
FUNCTION_BLOCK FB4

TITLE =   <CALCULO DE DESVIACION DE TEMPERATURAS DEL MOTOR>
//

AUTHOR:   H3       //
FAMILY:   DESV     //
NAME:     FB_DESV  //
VERSION:  01.00    //
// KNOW_HOW_PROTECT


VAR_INPUT
  NUM_CILINDROS : INT;
  Promedio      : REAL; 	// PROMEDIO DE LA TEMPERATURA DE LOS CILINDROS
  Lim_desv_alto : REAL;     // LIMITE DE DESVIACION ALTO
  Lim_desv_bajo : REAL;	    // LIMITE DE DESVIACION BAJO

END_VAR



VAR

  	TEMP_CIL1	: REAL;
  	TEMP_CIL2	: REAL;
  	TEMP_CIL3	: REAL;
  	TEMP_CIL4	: REAL;
  	TEMP_CIL5	: REAL;
  	TEMP_CIL6	: REAL;
  	TEMP_CIL7	: REAL;
  	TEMP_CIL8	: REAL;
  	TEMP_CIL9	: REAL;
  	TEMP_CIL10	: REAL;
  	TEMP_CIL11	: REAL;
  	TEMP_CIL12	: REAL;
  	TEMP_CIL13	: REAL;
  	TEMP_CIL14	: REAL;
  	TEMP_CIL15	: REAL;
  	TEMP_CIL16	: REAL;
  	TEMP_CIL17	: REAL;
  	TEMP_CIL18	: REAL;
  	TEMP_CIL19	: REAL;
	TEMP_CIL20	: REAL;


  	DEV_CIL1	: REAL;
  	DEV_CIL2	: REAL;
  	DEV_CIL3	: REAL;
  	DEV_CIL4	: REAL;
  	DEV_CIL5	: REAL;
  	DEV_CIL6	: REAL;
  	DEV_CIL7	: REAL;
  	DEV_CIL8	: REAL;
  	DEV_CIL9	: REAL;
  	DEV_CIL10	: REAL;
  	DEV_CIL11	: REAL;
  	DEV_CIL12	: REAL;
  	DEV_CIL13	: REAL;
  	DEV_CIL14	: REAL;
  	DEV_CIL15	: REAL;
  	DEV_CIL16	: REAL;
  	DEV_CIL17	: REAL;
  	DEV_CIL18	: REAL;
  	DEV_CIL19	: REAL;
	DEV_CIL20	: REAL;


	DEV_CIL1_AL		: BOOL;
  	DEV_CIL2_AL		: BOOL;
  	DEV_CIL3_AL		: BOOL;
  	DEV_CIL4_AL		: BOOL;
  	DEV_CIL5_AL		: BOOL;
  	DEV_CIL6_AL		: BOOL;
  	DEV_CIL7_AL		: BOOL;
  	DEV_CIL8_AL		: BOOL;
  	DEV_CIL9_AL		: BOOL;
  	DEV_CIL10_AL	: BOOL;
  	DEV_CIL11_AL	: BOOL;
  	DEV_CIL12_AL	: BOOL;
  	DEV_CIL13_AL	: BOOL;
  	DEV_CIL14_AL	: BOOL;
  	DEV_CIL15_AL	: BOOL;
  	DEV_CIL16_AL	: BOOL;
  	DEV_CIL17_AL	: BOOL;
  	DEV_CIL18_AL	: BOOL;
  	DEV_CIL19_AL	: BOOL;
	DEV_CIL20_AL	: BOOL;


	FallSen_CIL1	: BOOL;
  	FallSen_CIL2	: BOOL;
  	FallSen_CIL3	: BOOL;
  	FallSen_CIL4	: BOOL;
  	FallSen_CIL5	: BOOL;
  	FallSen_CIL6	: BOOL;
  	FallSen_CIL7	: BOOL;
  	FallSen_CIL8	: BOOL;
  	FallSen_CIL9	: BOOL;
  	FallSen_CIL10	: BOOL;
  	FallSen_CIL11	: BOOL;
  	FallSen_CIL12	: BOOL;
  	FallSen_CIL13	: BOOL;
  	FallSen_CIL14	: BOOL;
  	FallSen_CIL15	: BOOL;
  	FallSen_CIL16	: BOOL;
  	FallSen_CIL17	: BOOL;
  	FallSen_CIL18	: BOOL;
  	FallSen_CIL19	: BOOL;
	FallSen_CIL20	: BOOL;

  	suma_temp : real;
  	num_cilindros_temp	: INT;


END_VAR


BEGIN
NETWORK
TITLE =   <VERIFICANDO FALLAD DE SENSOR>
// CALCULA EL PROMEDIO DE TEMPERATURA TOMANDO EN CUENTA
// LOS CILINDROS QUE PRESENTAN PROBLEMAS DE SENSOR Y LOS ELIMINA DEL
// CALCULO.
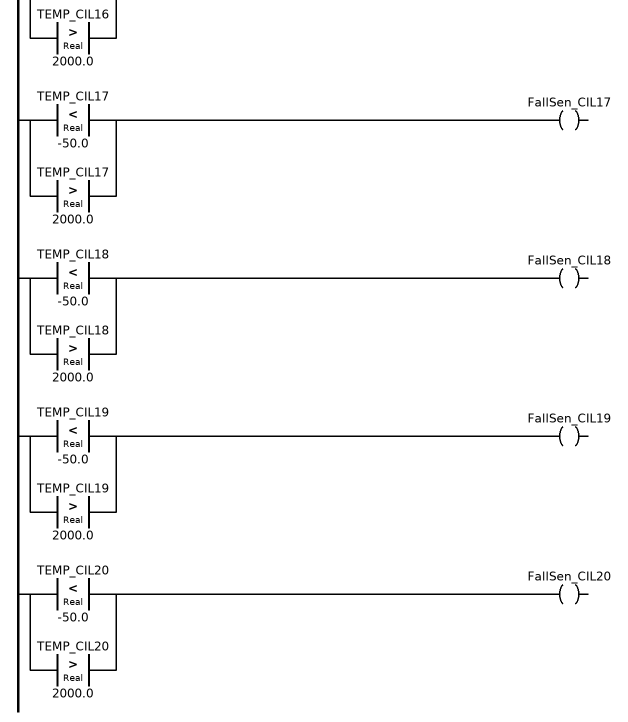
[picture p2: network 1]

	// Verificando falla de sensores
	O(;
	L TEMP_CIL1;
	L -50.0;
	<r;
	);
	o(;
	L TEMP_CIL1;
	L 2000.0;
	>r;
	);
	= FallSen_CIL1;

	O(;
	L TEMP_CIL2;
	L -50.0;
	<r;
	);
	o(;
	L TEMP_CIL2;
	L 2000.0;
	>r;
	);
	= FallSen_CIL2;

	O(;
	L TEMP_CIL3;
	L -50.0;
	<r;
	);
	o(;
	L TEMP_CIL3;
	L 2000.0;
	>r;
	);
	= FallSen_CIL3;


    O(;
	L TEMP_CIL4;
	L -50.0;
	<r;
	);
	o(;
	L TEMP_CIL4;
	L 2000.0;
	>r;
	);
	= FallSen_CIL4;

	O(;
	L TEMP_CIL4;
	L -50.0;
	<r;
	);
	o(;
	L TEMP_CIL4;
	L 2000.0;
	>r;
	);
	= FallSen_CIL4;


    O(;
	L TEMP_CIL5;
	L -50.0;
	<r;
	);
	o(;
	L TEMP_CIL5;
	L 2000.0;
	>r;
	);
	= FallSen_CIL5;


	O(;
	L TEMP_CIL6;
	L -50.0;
	<r;
	);
	o(;
	L TEMP_CIL6;
	L 2000.0;
	>r;
	);
	= FallSen_CIL6;


	O(;
	L TEMP_CIL7;
	L -50.0;
	<r;
	);
	o(;
	L TEMP_CIL7;
	L 2000.0;
	>r;
	);
	= FallSen_CIL7;


	O(;
	L TEMP_CIL8;
	L -50.0;
	<r;
	);
	o(;
	L TEMP_CIL8;
	L 2000.0;
	>r;
	);
	= FallSen_CIL8;

	O(;
	L TEMP_CIL9;
	L -50.0;
	<r;
	);
	o(;
	L TEMP_CIL9;
	L 2000.0;
	>r;
	);
	= FallSen_CIL9;


	O(;
	L TEMP_CIL10;
	L -50.0;
	<r;
	);
	o(;
	L TEMP_CIL10;
	L 2000.0;
	>r;
	);
	= FallSen_CIL10;


	O(;
	L TEMP_CIL11;
	L -50.0;
	<r;
	);
	o(;
	L TEMP_CIL11;
	L 2000.0;
	>r;
	);
	= FallSen_CIL11;

	O(;
	L TEMP_CIL12;
	L -50.0;
	<r;
	);
	o(;
	L TEMP_CIL12;
	L 2000.0;
	>r;
	);
	= FallSen_CIL12;


	O(;
	L TEMP_CIL13;
	L -50.0;
	<r;
	);
	o(;
	L TEMP_CIL13;
	L 2000.0;
	>r;
	);
	= FallSen_CIL13;


	O(;
	L TEMP_CIL14;
	L -50.0;
	<r;
	);
	o(;
	L TEMP_CIL14;
	L 2000.0;
	>r;
	);
	= FallSen_CIL14;


	O(;
	L TEMP_CIL15;
	L -50.0;
	<r;
	);
	o(;
	L TEMP_CIL15;
	L 2000.0;
	>r;
	);
	= FallSen_CIL15;


	O(;
	L TEMP_CIL16;
	L -50.0;
	<r;
	);
	o(;
	L TEMP_CIL16;
	L 2000.0;
	>r;
	);
	= FallSen_CIL16;


	O(;
	L TEMP_CIL17;
	L -50.0;
	<r;
	);
	o(;
	L TEMP_CIL17;
	L 2000.0;
	>r;
	);
	= FallSen_CIL17;


	O(;
	L TEMP_CIL18;
	L -50.0;
	<r;
	);
	o(;
	L TEMP_CIL18;
	L 2000.0;
	>r;
	);
	= FallSen_CIL18;


	O(;
	L TEMP_CIL19;
	L -50.0;
	<r;
	);
	o(;
	L TEMP_CIL19;
	L 2000.0;
	>r;
	);
	= FallSen_CIL19;

	O(;
	L TEMP_CIL20;
	L -50.0;
	<r;
	);
	o(;
	L TEMP_CIL20;
	L 2000.0;
	>r;
	);
	= FallSen_CIL20;

NETWORK
TITLE =   <CALCULA EL PROMEDIO DE LAS TEMPERATURAS>
// CALCULA EL PROMEDIO DE TEMPERATURA TOMANDO EN CUENTA

	L 0;
	T suma_temp;
  	L num_cilindros;
  	T num_cilindros_temp;


	L num_cilindros;
	L 1;
	<I;
	jc fin;

	AN FallSen_CIL1;
	jc cil1;

	L num_cilindros_temp;
	dec 1;
	T num_cilindros_temp;
	jc nxt2;

cil1:	L TEMP_CIL1;
	L suma_temp;
	+r;
	t suma_temp;


nxt2:	L num_cilindros;
	L 2;
	<I;
	jc fin;

	AN FallSen_CIL2;
	jc cil2;

	L num_cilindros_temp;
	dec 1;
	T num_cilindros_temp;
	jc nxt3;

cil2:	L TEMP_CIL2;
	L suma_temp;
	+r;
	t suma_temp;


nxt3:	L num_cilindros;
	L 3;
	<I;
	jc fin;

	AN FallSen_CIL3;
	jc cil3;

	L num_cilindros_temp;
	dec 1;
	T num_cilindros_temp;
	jc nxt4;

cil3:	L TEMP_CIL3;
	L suma_temp;
	+r;
	t suma_temp;


nxt4:	L num_cilindros;
	L 4;
	<I;
	jc fin;

	AN FallSen_CIL4;
	jc cil4;

	L num_cilindros_temp;
	dec 1;
	T num_cilindros_temp;
	jc nxt5;

cil4:	L TEMP_CIL4;
	L suma_temp;
	+r;
	t suma_temp;


nxt5:	L num_cilindros;
	L 5;
	<I;
	jc fin;

	AN FallSen_CIL5;
	jc cil5;

	L num_cilindros_temp;
	dec 1;
	T num_cilindros_temp;
	jc nxt6;

cil5:	L TEMP_CIL5;
	L suma_temp;
	+r;
	t suma_temp;


nxt6:	L num_cilindros;
	L 6;
	<I;
	jc fin;

	AN FallSen_CIL6;
	jc cil6;

	L num_cilindros_temp;
	dec 1;
	T num_cilindros_temp;
	jc nxt7;

cil6:	L TEMP_CIL6;
	L suma_temp;
	+r;
	t suma_temp;


nxt7:	L num_cilindros;
	L 7;
	<I;
	jc fin;

	AN FallSen_CIL7;
	jc cil7;

	L num_cilindros_temp;
	dec 1;
	T num_cilindros_temp;
	jc nxt8;

cil7:	L TEMP_CIL7;
	L suma_temp;
	+r;
	t suma_temp;


nxt8:	L num_cilindros;
	L 8;
	<I;
	jc fin;

	AN FallSen_CIL8;
	jc cil8;

	L num_cilindros_temp;
	dec 1;
	T num_cilindros_temp;
	jc nxt9;

cil8:	L TEMP_CIL8;
	L suma_temp;
	+r;
	t suma_temp;


nxt9:	L num_cilindros;
	L 9;
	<I;
	jc fin;

	AN FallSen_CIL9;
	jc cil9;

	L num_cilindros_temp;
	dec 1;
	T num_cilindros_temp;
	jc nx10;

cil9:	L TEMP_CIL9;
	L suma_temp;
	+r;
	t suma_temp;


nx10:	L num_cilindros;
	L 10;
	<I;
	jc fin;

	AN FallSen_CIL10;
	jc cl10;

	L num_cilindros_temp;
	dec 1;
	T num_cilindros_temp;
	jc nx11;

cl10:	L TEMP_CIL10;
	L suma_temp;
	+r;
	t suma_temp;


nx11:	L num_cilindros;
	L 11;
	<I;
	jc fin;

	AN FallSen_CIL11;
	jc cl11;

	L num_cilindros_temp;
	dec 1;
	T num_cilindros_temp;
	jc nx12;

cl11:	L TEMP_CIL11;
	L suma_temp;
	+r;
	t suma_temp;


nx12:	L num_cilindros;
	L 12;
	<I;
	jc fin;

	AN FallSen_CIL12;
	jc cl12;

	L num_cilindros_temp;
	dec 1;
	T num_cilindros_temp;
	jc nx13;

cl12:	L TEMP_CIL12;
	L suma_temp;
	+r;
	t suma_temp;


nx13:	L num_cilindros;
	L 13;
	<I;
	jc fin;

	AN FallSen_CIL13;
	jc cl13;

	L num_cilindros_temp;
	dec 1;
	T num_cilindros_temp;
	jc nx14;

cl13:	L TEMP_CIL13;
	L suma_temp;
	+r;
	t suma_temp;


nx14:	L num_cilindros;
	L 14;
	<I;
	jc fin;

	AN FallSen_CIL14;
	jc cl14;

	L num_cilindros_temp;
	dec 1;
	T num_cilindros_temp;
	jc nx15;

cl14:	L TEMP_CIL14;
	L suma_temp;
	+r;
	t suma_temp;


nx15:	L num_cilindros;
	L 15;
	<I;
	jc fin;

	AN FallSen_CIL15;
	jc cl15;

	L num_cilindros_temp;
	dec 1;
	T num_cilindros_temp;
	jc nx16;

cl15:	L TEMP_CIL15;
	L suma_temp;
	+r;
	t suma_temp;


nx16:	L num_cilindros;
	L 16;
	<I;
	jc fin;

	AN FallSen_CIL16;
	jc cl16;

	L num_cilindros_temp;
	dec 1;
	T num_cilindros_temp;
	jc nx17;

cl16:	L TEMP_CIL16;
	L suma_temp;
	+r;
	t suma_temp;


nx17:	L num_cilindros;
	L 17;
	<I;
	jc fin;

	AN FallSen_CIL17;
	jc cl17;

	L num_cilindros_temp;
	dec 1;
	T num_cilindros_temp;
	jc nx18;

cl17:	L TEMP_CIL17;
	L suma_temp;
	+r;
	t suma_temp;


nx18:	L num_cilindros;
	L 18;
	<I;
	jc fin;

	AN FallSen_CIL18;
	jc cl18;

	L num_cilindros_temp;
	dec 1;
	T num_cilindros_temp;
	jc nx19;

cl18:	L TEMP_CIL18;
	L suma_temp;
	+r;
	t suma_temp;


nx19:	L num_cilindros;
	L 19;
	<I;
	jc fin;

	AN FallSen_CIL19;
	jc cl19;

	L num_cilindros_temp;
	dec 1;
	T num_cilindros_temp;
	jc nx20;

cl19:	L TEMP_CIL19;
	L suma_temp;
	+r;
	t suma_temp;


nx20:	L num_cilindros;
	L 20;
	<I;
	jc fin;

	AN FallSen_CIL20;
	jc cl20;

	L num_cilindros_temp;
	dec 1;
	T num_cilindros_temp;
	jc fin;

cl20:	L TEMP_CIL20;
	L suma_temp;
	+r;
	t suma_temp;




fin : nop 0;

	L suma_temp;
  	L num_cilindros_temp;
  	itd;
  	dtr;
  	/r;
  	t promedio;

NETWORK
TITLE =   <CALCULA LA DESVIACION DE CADA CILINDRO>
// DESVIACION DE CILINDRO = TEMPERATURA DE CILINDRO - PROMEDIO

	L num_cilindros;
	L 1;
	>=I;
	JC DV1;
	L 0;
	T DEV_CIL1;
	ju fin2;

DV1:	L TEMP_CIL1;
	L PROMEDIO;
	-R;
	T DEV_CIL1;


	L num_cilindros;
	L 2;
	>=I;
	JC DV2;
	L 0;
	T DEV_CIL2;
	ju fin2;

DV2:	L TEMP_CIL2;
	L PROMEDIO;
	-R;
	T DEV_CIL2;


	L num_cilindros;
	L 3;
	>=I;
	JC DV3;
	L 0;
	T DEV_CIL3;
	ju fin2;
DV3:	L TEMP_CIL3;
	L PROMEDIO;
	-R;
	T DEV_CIL3;

	L num_cilindros;
	L 4;
	>=I;
	JC DV4;
	L 0;
	T DEV_CIL4;
	ju fin2;
DV4:	L TEMP_CIL4;
	L PROMEDIO;
	-R;
	T DEV_CIL4;

	L num_cilindros;
	L 5;
	>=I;
	JC DV5;
	L 0;
	T DEV_CIL5;
	ju fin2;
DV5:	L TEMP_CIL5;
	L PROMEDIO;
	-R;
	T DEV_CIL5;

	L num_cilindros;
	L 6;
	>=I;
	JC DV6;
	L 0;
	T DEV_CIL6;
	ju fin2;
DV6:	L TEMP_CIL6;
	L PROMEDIO;
	-R;
	T DEV_CIL6;

	L num_cilindros;
	L 7;
	>=I;
	JC DV7;
	L 0;
	T DEV_CIL7;
	ju fin2;
DV7:	L TEMP_CIL7;
	L PROMEDIO;
	-R;
	T DEV_CIL7;

	L num_cilindros;
	L 8;
	>=I;
	JC DV8;
	L 0;
	T DEV_CIL8;
	ju fin2;
DV8:	L TEMP_CIL8;
	L PROMEDIO;
	-R;
	T DEV_CIL8;


	L num_cilindros;
	L 9;
	>=I;
	JC DV9;
	L 0;
	T DEV_CIL9;
	ju fin2;
DV9:	L TEMP_CIL9;
	L PROMEDIO;
	-R;
	T DEV_CIL9;


	L num_cilindros;
	L 10;
	>=I;
	JC DV10;
	L 0;
	T DEV_CIL10;
	ju fin2;
DV10:	L TEMP_CIL10;
	L PROMEDIO;
	-R;
	T DEV_CIL10;

	L num_cilindros;
	L 11;
	>=I;
	JC DV11;
	L 0;
	T DEV_CIL11;
	ju fin2;
DV11:	L TEMP_CIL11;
	L PROMEDIO;
	-R;
	T DEV_CIL11;


	L num_cilindros;
	L 12;
	>=I;
	JC DV12;
	L 0;
	T DEV_CIL12;
	ju fin2;
DV12:	L TEMP_CIL12;
	L PROMEDIO;
	-R;
	T DEV_CIL12;

	L num_cilindros;
	L 13;
	>=I;
	JC DV13;
	L 0;
	T DEV_CIL13;
	ju fin2;
DV13:	L TEMP_CIL13;
	L PROMEDIO;
	-R;
	T DEV_CIL13;

	L num_cilindros;
	L 14;
	>=I;
	JC DV14;
	L 0;
	T DEV_CIL14;
	ju fin2;
DV14:	L TEMP_CIL14;
	L PROMEDIO;
	-R;
	T DEV_CIL14;


	L num_cilindros;
	L 15;
	>=I;
	JC DV15;
	L 0;
	T DEV_CIL15;
	ju fin2;
DV15:	L TEMP_CIL15;
	L PROMEDIO;
	-R;
	T DEV_CIL15;

	L num_cilindros;
	L 16;
	>=I;
	JC DV16;
	L 0;
	T DEV_CIL16;
	ju fin2;
DV16:	L TEMP_CIL16;
	L PROMEDIO;
	-R;
	T DEV_CIL16;

	L num_cilindros;
	L 17;
	>=I;
	JC DV17;
	L 0;
	T DEV_CIL17;
	ju fin2;
DV17:	L TEMP_CIL17;
	L PROMEDIO;
	-R;
	T DEV_CIL17;

	L num_cilindros;
	L 18;
	>=I;
	JC DV18;
	L 0;
	T DEV_CIL18;
	ju fin2;
DV18:	L TEMP_CIL18;
	L PROMEDIO;
	-R;
	T DEV_CIL18;

	L num_cilindros;
	L 19;
	>=I;
	JC DV19;
	L 0;
	T DEV_CIL19;
	ju fin2;
DV19:	L TEMP_CIL19;
	L PROMEDIO;
	-R;
	T DEV_CIL19;

	L num_cilindros;
	L 20;
	>=I;
	JC DV20;
	L 0;
	T DEV_CIL20;
	ju fin2;
DV20:	L TEMP_CIL20;
	L PROMEDIO;
	-R;
	T DEV_CIL20;


fin2: nop 0;


NETWORK
TITLE =   <FALLA DE DESVIACION>
// DESVIACION DE CILINDRO > Lim_desv_alto O DESVIACION DE CILINDRO > Lim_desv_BAJO
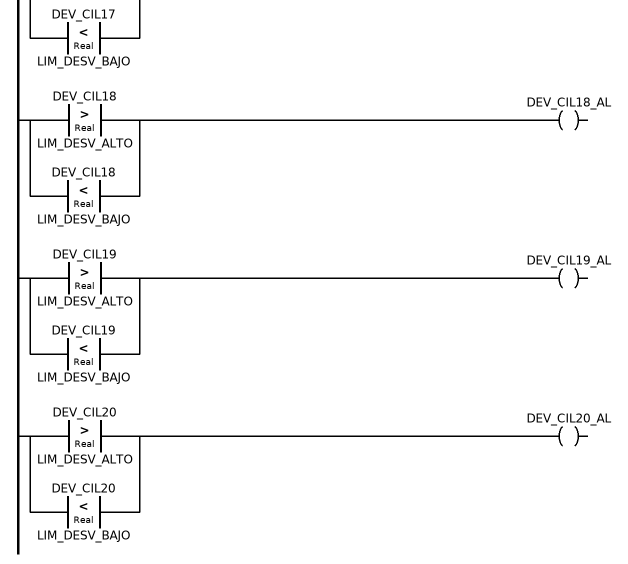
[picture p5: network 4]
	O(;
	L DEV_CIL1;
	L LIM_DESV_ALTO;
	>R;
	);
	O(;
	L DEV_CIL1;
	L LIM_DESV_BAJO;
	<R;
	);
	= DEV_CIL1_AL;

	O(;
	L DEV_CIL2;
	L LIM_DESV_ALTO;
	>R;
	);
	O(;
	L DEV_CIL2;
	L LIM_DESV_BAJO;
	<R;
	);
	= DEV_CIL2_AL;

	O(;
	L DEV_CIL3;
	L LIM_DESV_ALTO;
	>R;
	);
	O(;
	L DEV_CIL3;
	L LIM_DESV_BAJO;
	<R;
	);
	= DEV_CIL3_AL;

	O(;
	L DEV_CIL4;
	L LIM_DESV_ALTO;
	>R;
	);
	O(;
	L DEV_CIL4;
	L LIM_DESV_BAJO;
	<R;
	);
	= DEV_CIL4_AL;

	O(;
	L DEV_CIL5;
	L LIM_DESV_ALTO;
	>R;
	);
	O(;
	L DEV_CIL5;
	L LIM_DESV_BAJO;
	<R;
	);
	= DEV_CIL5_AL;

	O(;
	L DEV_CIL6;
	L LIM_DESV_ALTO;
	>R;
	);
	O(;
	L DEV_CIL6;
	L LIM_DESV_BAJO;
	<R;
	);
	= DEV_CIL6_AL;

  	O(;
	L DEV_CIL7;
	L LIM_DESV_ALTO;
	>R;
	);
	O(;
	L DEV_CIL7;
	L LIM_DESV_BAJO;
	<R;
	);
	= DEV_CIL7_AL;

	O(;
	L DEV_CIL8;
	L LIM_DESV_ALTO;
	>R;
	);
	O(;
	L DEV_CIL8;
	L LIM_DESV_BAJO;
	<R;
	);
	= DEV_CIL8_AL;

	O(;
	L DEV_CIL9;
	L LIM_DESV_ALTO;
	>R;
	);
	O(;
	L DEV_CIL9;
	L LIM_DESV_BAJO;
	<R;
	);
	= DEV_CIL9_AL;

	O(;
	L DEV_CIL10;
	L LIM_DESV_ALTO;
	>R;
	);
	O(;
	L DEV_CIL10;
	L LIM_DESV_BAJO;
	<R;
	);
	= DEV_CIL10_AL;

	O(;
	L DEV_CIL11;
	L LIM_DESV_ALTO;
	>R;
	);
	O(;
	L DEV_CIL11;
	L LIM_DESV_BAJO;
	<R;
	);
	= DEV_CIL11_AL;

	O(;
	L DEV_CIL12;
	L LIM_DESV_ALTO;
	>R;
	);
	O(;
	L DEV_CIL12;
	L LIM_DESV_BAJO;
	<R;
	);
	= DEV_CIL12_AL;

	O(;
	L DEV_CIL13;
	L LIM_DESV_ALTO;
	>R;
	);
	O(;
	L DEV_CIL13;
	L LIM_DESV_BAJO;
	<R;
	);
	= DEV_CIL13_AL;

	O(;
	L DEV_CIL14;
	L LIM_DESV_ALTO;
	>R;
	);
	O(;
	L DEV_CIL14;
	L LIM_DESV_BAJO;
	<R;
	);
	= DEV_CIL14_AL;

	O(;
	L DEV_CIL15;
	L LIM_DESV_ALTO;
	>R;
	);
	O(;
	L DEV_CIL15;
	L LIM_DESV_BAJO;
	<R;
	);
	= DEV_CIL15_AL;

	O(;
	L DEV_CIL16;
	L LIM_DESV_ALTO;
	>R;
	);
	O(;
	L DEV_CIL16;
	L LIM_DESV_BAJO;
	<R;
	);
	= DEV_CIL16_AL;

	O(;
	L DEV_CIL17;
	L LIM_DESV_ALTO;
	>R;
	);
	O(;
	L DEV_CIL17;
	L LIM_DESV_BAJO;
	<R;
	);
	= DEV_CIL17_AL;

	O(;
	L DEV_CIL18;
	L LIM_DESV_ALTO;
	>R;
	);
	O(;
	L DEV_CIL18;
	L LIM_DESV_BAJO;
	<R;
	);
	= DEV_CIL18_AL;

	O(;
	L DEV_CIL19;
	L LIM_DESV_ALTO;
	>R;
	);
	O(;
	L DEV_CIL19;
	L LIM_DESV_BAJO;
	<R;
	);
	= DEV_CIL19_AL;

	O(;
	L DEV_CIL20;
	L LIM_DESV_ALTO;
	>R;
	);
	O(;
	L DEV_CIL20;
	L LIM_DESV_BAJO;
	<R;
	);
	= DEV_CIL20_AL;


END_FUNCTION_BLOCK



